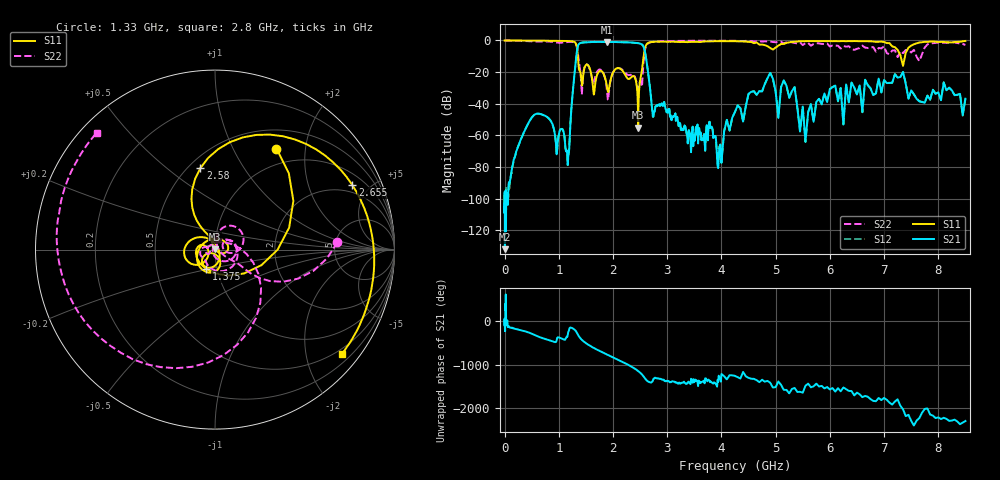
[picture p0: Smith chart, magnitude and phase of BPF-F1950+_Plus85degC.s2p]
! Mini-Circuits
! S2P DATA File Format
! Type: BAND PASS FILTER
! Model: BPF-F1950+
! All S Parameters are in dB deg format
! TEST CONDITIONS: INPUT POWER = 0 dBm @ Temperature = +85deg C
# MHz S dB R 50
!Frequency  S11 dB  S11 DEG  S21 dB  S21 DEG  S12 dB  S12 DEG  S22 dB  S22 DEG
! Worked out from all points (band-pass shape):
!   712 points, 1 MHz to 8.5 GHz, reference 50 ohm
!   highest |S21| = -0.90 dB at 1.885 GHz (marker M1); lowest = -131.9 dB at 6 MHz (marker M2)
!   |S21| within 3 dB of the highest: 1.35 GHz to 2.564 GHz (1.214 GHz wide, 62 % of centre)
!   lowest |S11| = -55.2 dB at 2.465 GHz (marker M3), VSWR 1.00, Z = 50.1 + j0.137 ohm
!   |S11| at or under -10 dB: 1.352 GHz to 2.566 GHz (1.214 GHz wide, 62 % of centre); 7.306 GHz to 7.386 GHz (80.72 MHz wide, 1.1 % of centre)
!   |S22| runs from -37.7 to 0.0 dB; largest |S21 - S12| = 0.0019
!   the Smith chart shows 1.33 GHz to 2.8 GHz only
!   S11 on the Smith chart (normalised r, x): 1.33 GHz: 0.75, +1.50; 1.375 GHz: 0.88, -0.19; 2.58 GHz: 0.57, +0.66; 2.655 GHz: 1.54, +3.89; 2.8 GHz: 0.38, -2.73
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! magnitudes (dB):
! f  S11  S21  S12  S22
! 1 MHz  0.0  -103.0  -95.9  0.0
! 6 MHz  0.0  -131.9  -98.1  0.0
! 600 MHz  -0.1  -46.3  -46.3  -0.7
! 1.175 GHz  -0.4  -73.1  -73.7  -0.9
! 1.33 GHz  -3.6  -8.0  -8.0  -3.3
! 1.375 GHz  -18.5  -2.1  -2.1  -14.7
! 1.42 GHz  -25.9  -1.4  -1.4  -31.0
! 1.515 GHz  -15.2  -1.2  -1.2  -15.1
! 1.885 GHz  -28.4  -0.9  -0.9  -30.3
! 2.135 GHz  -17.9  -1.1  -1.1  -17.7
! 2.465 GHz  -55.2  -1.7  -1.7  -30.8
! 2.58 GHz  -6.7  -5.6  -5.6  -8.2
! 2.655 GHz  -1.5  -22.3  -22.3  -1.6
! 2.8 GHz  -0.8  -41.3  -41.3  -0.7
! 2.835 GHz  -0.7  -40.7  -40.7  -0.6
! 3.81 GHz  -0.5  -54.6  -54.7  -0.2
! 3.94 GHz  -0.5  -80.7  -79.4  -0.2
! 4.3 GHz  -0.5  -41.0  -41.0  -0.3
! 4.85 GHz  -3.6  -23.8  -23.8  -0.6
! 5.7 GHz  -0.4  -51.4  -51.3  -2.3
! 7.1 GHz  -1.7  -26.9  -26.8  -8.7
! 8.5 GHz  -0.3  -36.9  -36.8  -2.9
